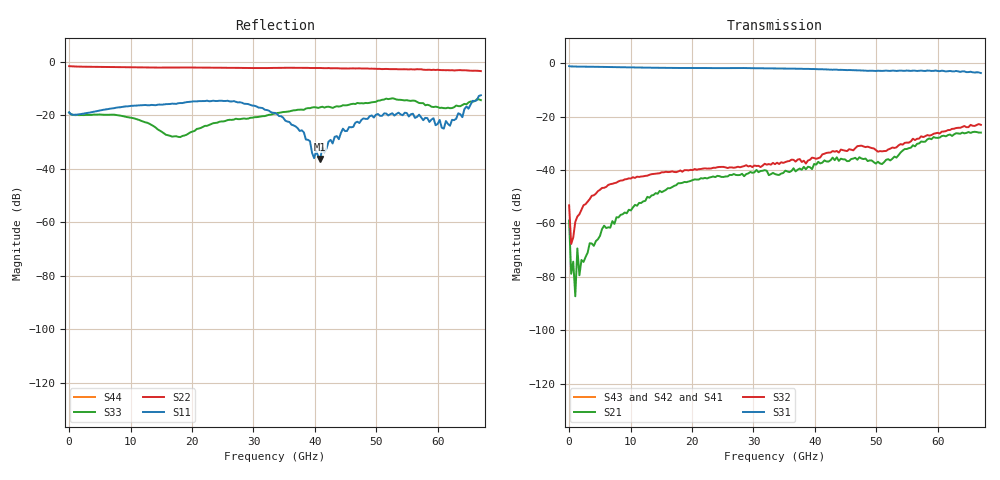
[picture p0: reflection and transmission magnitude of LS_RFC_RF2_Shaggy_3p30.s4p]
!Keysight Technologies,N5227A,US51270237,A.10.65.04
!Date: Wednesday, April 27, 2022 16:37:02
!Correction: S11(Full 3 Port(1,2,3))
!S12(Full 3 Port(1,2,3))
!S13(Full 3 Port(1,2,3))
!S14(Off)
!S21(Full 3 Port(1,2,3))
!S22(Full 3 Port(1,2,3))
!S23(Full 3 Port(1,2,3))
!S24(Off)
!S31(Full 3 Port(1,2,3))
!S32(Full 3 Port(1,2,3))
!S33(Full 3 Port(1,2,3))
!S34(Off)
!S41(Off)
!S42(Off)
!S43(Off)
!S44(Off)
!S4P File: Measurements: <S11,S12,S13,S14>,
!<S21,S22,S23,S24>,
!<S31,S32,S33,S34>,
!<S41,S42,S43,S44>:
# Hz S  dB  R 50
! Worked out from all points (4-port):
!   201 points, 10 MHz to 67 GHz, reference 50 ohm
!   strongest paths, dB at 10 MHz, 16.76 GHz, 33.51 GHz, 50.25 GHz, 67 GHz:
!     S31: -1.1, -1.8, -2.0, -2.8, -3.7
!     S32: -53.2, -40.5, -37.8, -33.1, -23.1
!     S21: -58.9, -46.4, -41.5, -36.9, -26.0
!     S43: -, -, -, -, -
!     S42: -, -, -, -, -
!     S41: -, -, -, -, -
!   lowest |S11| = -36.3 dB at 40.87 GHz (marker M1), VSWR 1.03, Z = 48.7 + j0.731 ohm
!   |S11| at or under -10 dB: start of sweep to end of sweep
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1e7  -18.81 -1.7  -62.15 -82.2  -1.11 -0.1  -200.00 45.0
     -58.92 132.4  -1.53 179.9  -51.84 179.6  -200.00 45.0
     -1.12 -0.2  -53.23 -133.5  -18.93 -1.0  -200.00 45.0
     -200.00 45.0  -200.00 45.0  -200.00 45.0  -200.00 45.0
3.4495e8  -19.56 -7.1  -83.63 -149.3  -1.23 -3.4  -200.00 45.0
          -78.89 52.1  -1.58 177.5  -72.62 130.2  -200.00 45.0
          -1.21 -3.4  -67.71 70.7  -19.60 -6.9  -200.00 45.0
          -200.00 45.0  -200.00 45.0  -200.00 45.0  -200.00 45.0
1.01485e9  -19.68 -15.6  -80.04 -64.7  -1.27 -9.0  -200.00 45.0
           -87.30 150.6  -1.66 173.7  -62.11 75.2  -200.00 45.0
           -1.26 -9.0  -59.44 64.3  -19.86 -15.3  -200.00 45.0
           -200.00 45.0  -200.00 45.0  -200.00 45.0  -200.00 45.0
2.14468e10  -14.62 -156.2  -43.44 21.5  -1.84 -177.4  -200.00 45.0
            -43.09 22.5  -2.07 61.7  -39.86 -60.7  -200.00 45.0
            -1.81 -177.5  -39.63 -59.1  -24.65 -138.6  -200.00 45.0
            -200.00 45.0  -200.00 45.0  -200.00 45.0  -200.00 45.0
4.08739e10  -36.32 150.5  -37.34 -127.6  -2.26 18.0  -200.00 45.0
            -37.53 -131.0  -2.21 -33.0  -34.65 -168.6  -200.00 45.0
            -2.26 18.1  -35.28 -174.1  -16.91 18.0  -200.00 45.0
            -200.00 45.0  -200.00 45.0  -200.00 45.0  -200.00 45.0
5.393695e10  -19.56 33.0  -33.50 151.1  -2.76 -92.4  -200.00 45.0
             -33.46 153.9  -2.68 -96.2  -30.35 110.8  -200.00 45.0
             -2.77 -92.7  -30.29 112.2  -14.13 -74.9  -200.00 45.0
             -200.00 45.0  -200.00 45.0  -200.00 45.0  -200.00 45.0
6.7e10  -12.43 28.2  -26.04 41.8  -3.75 144.1  -200.00 45.0
        -25.99 43.3  -3.38 -172.3  -22.71 12.6  -200.00 45.0
        -3.69 143.7  -23.09 10.1  -14.25 74.7  -200.00 45.0
        -200.00 45.0  -200.00 45.0  -200.00 45.0  -200.00 45.0
